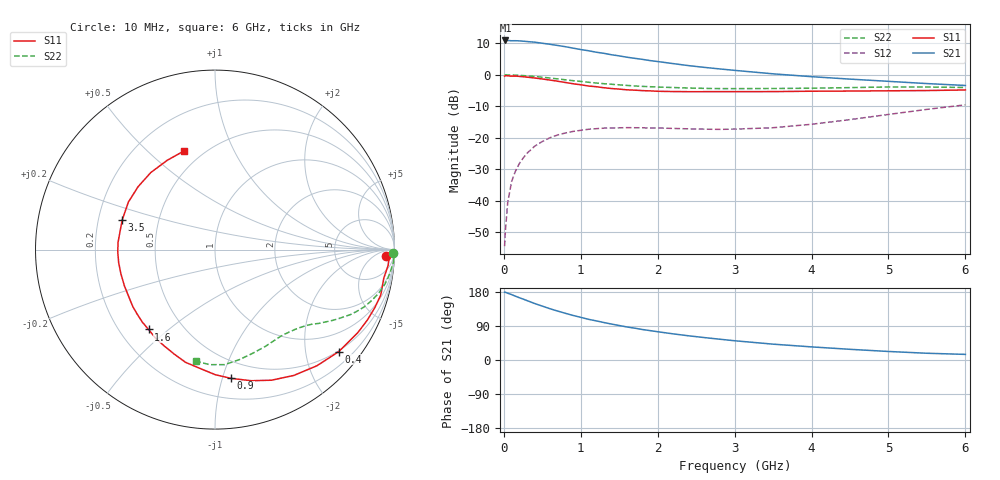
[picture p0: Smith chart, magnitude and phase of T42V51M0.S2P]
! Infineon Technologies  Discrete & RF Semiconductors
! BFR182T
! Si NPN RF Bipolar Junction Transistor in SC75
! VCE = 2.5 V  IC = 1 mA
! Common Emitter S-Parameters:  October  1999
# GHz  S  MA  R  50
!  f  S11  S21  S12  S22
! GHz  MAG  ANG  MAG  ANG  MAG  ANG  MAG  ANG
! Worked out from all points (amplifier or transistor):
!   36 points, 10 MHz to 6 GHz, reference 50 ohm
!   highest |S21| = 10.9 dB at 20 MHz (marker M1)
!   |S21| within 3 dB of that: start of sweep to 1.03 GHz
!   unconditionally stable (mu >= 1): 2.376 GHz to 4.583 GHz
!   at 250 MHz: K = 0.09, MSG = 18.6 dB, |S12| = -26.5 dB
!   at 1.4 GHz: K = 0.58, MSG = 11.6 dB, |S12| = -16.9 dB
!   at 6 GHz: K = 0.84, MSG = 3.1 dB, |S12| = -9.5 dB
!   S11 on the Smith chart (normalised r, x): 10 MHz: 27, -21; 400 MHz: 0.48, -2.71; 900 MHz: 0.36, -1.07; 1.6 GHz: 0.32, -0.43; 3.5 GHz: 0.30, +0.14; 6 GHz: 0.40, +0.66
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0.01  0.9545 -2.1  3.495 178.8  0.0019 85.7  0.9915 -1.1
0.02  0.9743 -0.8  3.525 178.8  0.0033 86.5  0.9999 -0.8
0.05  0.9686 -5.2  3.522 176.2  0.0093 87.5  0.9975 -2.0
0.1  0.9538 -9.6  3.487 172.7  0.02 85.3  0.9965 -4.0
0.2  0.9471 -20.1  3.471 164.5  0.0388 79.2  0.9831 -7.8
0.25  0.9353 -24.8  3.436 160.8  0.0475 75.2  0.9748 -9.6
0.4  0.8936 -39.5  3.31 149.1  0.0735 66.7  0.9439 -14.9
0.5  0.8611 -48.7  3.185 142.2  0.0874 62.1  0.918 -18.0
0.6  0.8274 -57.9  3.064 135.3  0.1004 57.2  0.8915 -20.9
0.7  0.7929 -66.6  2.934 129.1  0.1111 53.3  0.8634 -23.4
0.8  0.7578 -74.6  2.805 123.2  0.1193 49.6  0.836 -25.7
0.9  0.723 -82.9  2.663 117.6  0.1264 45.9  0.8092 -27.6
1.1  0.666 -97.6  2.42 107.4  0.1368 40.3  0.7639 -31.1
1.4  0.6072 -117.6  2.089 94.8  0.1433 34.0  0.7098 -35.4
1.6  0.5787 -129.8  1.909 87.2  0.1453 31.5  0.6803 -37.7
1.8  0.5627 -140.8  1.767 80.5  0.1446 30.0  0.6573 -40.3
2.2  0.5437 -158.1  1.512 69.0  0.1411 29.5  0.6299 -44.9
2.8  0.5418 -178.7  1.246 55.0  0.1363 34.1  0.6058 -53.1
3.5  0.5427 162.4  1.04 41.8  0.1448 45.3  0.6079 -62.6
4.5  0.5536 140.7  0.857 28.2  0.1947 58.0  0.6278 -77.5
5.5  0.5642 118.2  0.728 17.8  0.2832 59.7  0.6418 -92.6
6  0.5762 107.4  0.679 14.8  0.3344 56.9  0.6308 -99.7
